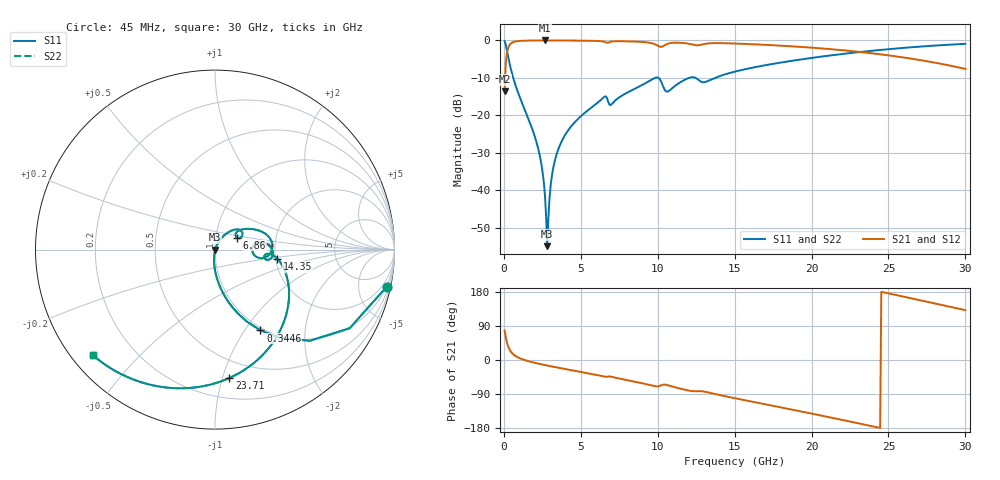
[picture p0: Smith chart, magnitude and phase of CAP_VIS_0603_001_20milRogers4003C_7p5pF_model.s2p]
! S-parameter model data by Modelithics Inc.  support@modelithics.com  813-866-6335  Tampa FL USA
! S-Parameter data specifications:
! Substrate: 20-mil Rogers 4003C, substrate thickness, H=0.508mm, Dielectric constant, Er=3.75
! PCB Mounting Pad Footprint: Pad width, PadW=0.90mm , Pad length, PadL=1.00mm , Pad gap, PadG (edge-to-edge)=1.00mm , Reference planes=3.0mm apart
! Created Wed Nov 18 13:24:55 2015
# hz S ma R 50
! 2 Port Network Data from SP1.SP block
! freq  magS11  angS11  magS21  angS21  magS12  angS12  magS22  angS22
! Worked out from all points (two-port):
!   401 points, 45 MHz to 30 GHz, reference 50 ohm
!   highest |S21| = -0.02 dB at 2.666 GHz (marker M1); lowest = -13.6 dB at 45 MHz (marker M2)
!   |S21| within 3 dB of the highest: 214.1 MHz to 23 GHz (22.78 GHz wide, 196 % of centre)
!   lowest |S11| = -54.9 dB at 2.816 GHz (marker M3), VSWR 1.00, Z = 50.2 - j0.064 ohm
!   |S11| at or under -10 dB: 604.9 MHz to 9.821 GHz (9.216 GHz wide, 177 % of centre); 10.05 GHz to 12.03 GHz (1.986 GHz wide, 18 % of centre); 12.46 GHz to 13.73 GHz (1.267 GHz wide, 9.67 % of centre)
!   |S22| runs from -54.9 to -0.2 dB; largest |S21 - S12| = 0
!   S11 on the Smith chart (normalised r, x): 45 MHz: 0.96, -9.20; 344.6 MHz: 0.96, -1.18; 6.86 GHz: 1.26, +0.17; 14.35 GHz: 2.05, -0.24; 23.71 GHz: 0.35, -1.05; 30 GHz: 0.06, -0.37
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4.5e7  0.978 -12.3  0.2086 77.7  0.2086 77.7  0.978 -12.3
3.4455e8  0.5165 -60.6  0.8557 29.3  0.8557 29.3  0.5165 -60.6
7.93875e8  0.238 -80.1  0.9703 9.6  0.9703 9.6  0.238 -80.1
2.216738e9  0.03682 -96.9  0.9975 -9.4  0.9975 -9.4  0.03682 -96.9
2.516288e9  0.01743 -96.5  0.9979 -12.1  0.9979 -12.1  0.01743 -96.5
2.666062e9  0.008709 -91.8  0.998 -13.4  0.998 -13.4  0.008709 -91.8
2.815838e9  0.001807 -20.7  0.998 -14.6  0.998 -14.6  0.001807 -20.7
2.965612e9  0.007973 60.7  0.9979 -15.9  0.9979 -15.9  0.007973 60.7
3.190275e9  0.01916 66.6  0.9976 -17.7  0.9976 -17.7  0.01916 66.6
3.489825e9  0.03333 66.5  0.9971 -20.0  0.9971 -20.0  0.03333 66.5
5.062462e9  0.1001 56.4  0.9917 -32.0  0.9917 -32.0  0.1001 56.4
6.485325e9  0.1744 39.4  0.9632 -43.6  0.9632 -43.6  0.1744 39.4
6.859762e9  0.1387 28.6  0.9473 -43.2  0.9473 -43.2  0.1387 28.6
9.0315e9  0.2572 25.2  0.9523 -61.8  0.9523 -61.8  0.2572 25.2
1.007992e10  0.3134 -2.6  0.8319 -69.1  0.8319 -69.1  0.3134 -2.6
1.067902e10  0.2092 2.9  0.9071 -66.8  0.9071 -66.8  0.2092 2.9
1.434851e10  0.3513 -8.3  0.9169 -95.4  0.9169 -95.4  0.3513 -8.3
1.50225e10  0.3838 -13.1  0.9081 -101.0  0.9081 -101.0  0.3838 -13.1
2.003996e10  0.5854 -52.6  0.7991 -141.7  0.7991 -141.7  0.5854 -52.6
2.370945e10  0.7197 -83.6  0.6809 -172.8  0.6809 -172.8  0.7197 -83.6
2.505742e10  0.7653 -95.4  0.6295 175.4  0.6295 175.4  0.7653 -95.4
3e10  0.8999 -139.2  0.4165 131.6  0.4165 131.6  0.8999 -139.2
